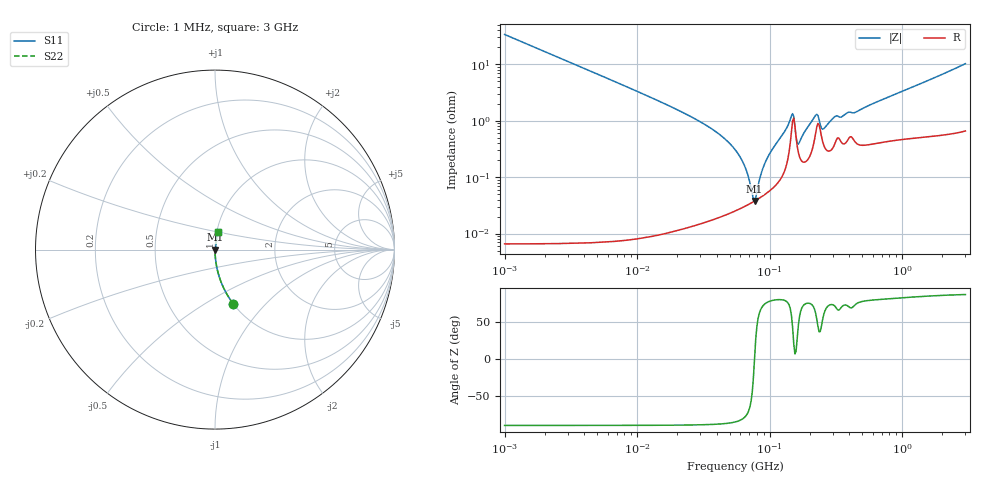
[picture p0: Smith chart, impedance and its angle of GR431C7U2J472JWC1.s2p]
!Murata Part Number: GR431C7U2J472JWC1
!These Parameters are Measured in Series Mode Connection
!Data Generated on Jun 10, 2025
!  o--ll--o
!Port1  Port2
!  o------o
!Operation Temp=25[degC], DC Bias Voltage=0[V]
!Freq. Start=1000[kHz] Stop=3[GHz] 401[Steps]
# Hz S RI R 50
!Freq.(Hz) S11(Real) S11(Imag) S21(Real) S21(Imag) S12(Real) S12(Imag) S22(Real) S22(Imag)
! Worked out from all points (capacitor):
!   401 points, 1 MHz to 3 GHz, reference 50 ohm
!   read as one part in series: C = 4.73 nF near 1.041 MHz
!   lowest |Z| = 37.6 mohm at 76.97 MHz (marker M1)
!   series resonance near 76.89 MHz, so ESL is about 910 pH
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1000000  0.1018 -0.3023  0.8982 0.3023  0.8982 0.3023  0.1018 -0.3023
3823119  0.00772 -0.0872  0.9923 0.0872  0.9923 0.0872  0.00772 -0.0872
1.461624e7  0.000586 -0.0222  0.9994 0.0222  0.9994 0.0222  0.000586 -0.0222
3.456417e7  0.000226 -0.00779  0.9998 0.00779  0.9998 0.00779  0.000226 -0.00779
5.477226e7  0.000259 -0.00307  0.9997 0.00307  0.9997 0.00307  0.000259 -0.00307
6.428402e7  0.000301 -0.00161  0.9997 0.00161  0.9997 0.00161  0.000301 -0.00161
6.826239e7  0.000322 -0.00107  0.9997 0.00107  0.9997 0.00107  0.000322 -0.00107
7.395247e7  0.000356 -0.000352  0.9996 0.000352  0.9996 0.000352  0.000356 -0.000352
7.697298e7  0.000376 1.03e-05  0.9996 -1.03e-05  0.9996 -1.03e-05  0.000376 1.03e-05
8.011685e7  0.000398 0.000376  0.9996 -0.000376  0.9996 -0.000376  0.000398 0.000376
8.679508e7  0.000449 0.00112  0.9996 -0.00112  0.9996 -0.00112  0.000449 0.00112
9.402997e7  0.000514 0.0019  0.9995 -0.0019  0.9995 -0.0019  0.000514 0.0019
1.460522e8  0.00643 0.0102  0.9936 -0.0102  0.9936 -0.0102  0.00643 0.0102
1.520175e8  0.011 0.00396  0.989 -0.00396  0.989 -0.00396  0.011 0.00396
1.646891e8  0.00273 0.00269  0.9973 -0.00269  0.9973 -0.00269  0.00273 0.00269
2.094008e8  0.00313 0.00948  0.9969 -0.00948  0.9969 -0.00948  0.00313 0.00948
2.268557e8  0.00779 0.0102  0.9922 -0.0102  0.9922 -0.0102  0.00779 0.0102
2.558035e8  0.00372 0.00612  0.9963 -0.00612  0.9963 -0.00612  0.00372 0.00612
3.124888e8  0.00415 0.0111  0.9959 -0.0111  0.9959 -0.0111  0.00415 0.0111
4.480278e8  0.00421 0.0135  0.9958 -0.0135  0.9958 -0.0135  0.00421 0.0135
8.005644e8  0.00498 0.026  0.995 -0.026  0.995 -0.026  0.00498 0.026
3e9  0.0166 0.0997  0.9834 -0.0997  0.9834 -0.0997  0.0166 0.0997
